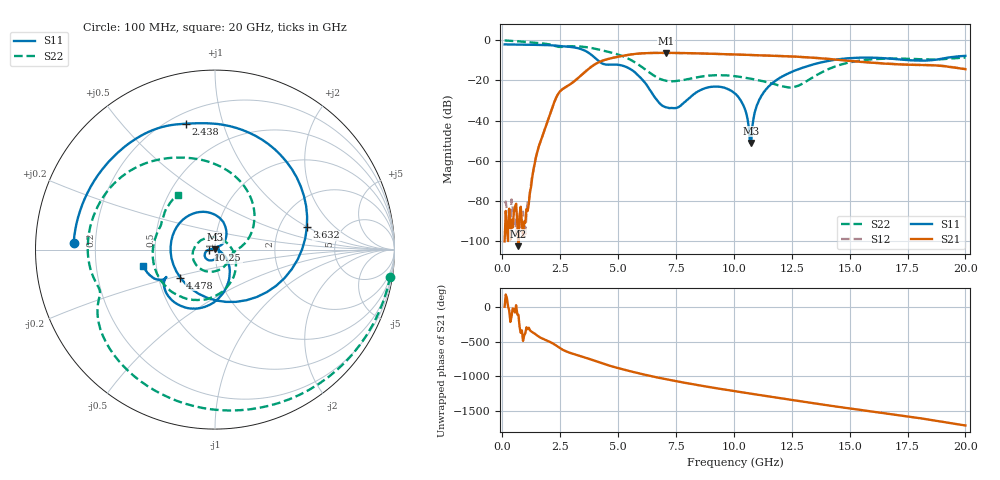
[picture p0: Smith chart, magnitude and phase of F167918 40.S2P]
!  2-Port S-parameters saved by WinCal
! VAR MeasName=S-Parameters (CALIBRATED_DATA) read from VNA (N5242A)
! VAR MeasDate=2016-11-22 10:26:40
! VAR NAME=F167918 40
! VAR FILENAME=F167918 40.S2P
! VAR DATE=2016-11-22 10:26:40
! VAR PHYS_PORTS=1,2
# Hz S DB R 50
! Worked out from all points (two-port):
!   401 points, 100 MHz to 20 GHz, reference 50 ohm
!   highest |S21| = -6.27 dB at 7.065 GHz (marker M1); lowest = -102.4 dB at 697 MHz (marker M2)
!   |S21| within 3 dB of the highest: 4.585 GHz to 14.08 GHz (9.496 GHz wide, 102 % of centre)
!   lowest |S11| = -51.1 dB at 10.75 GHz (marker M3), VSWR 1.01, Z = 50.2 + j0.14 ohm
!   |S11| at or under -10 dB: 4.123 GHz to 14.21 GHz (10.09 GHz wide, 110 % of centre); 17.69 GHz to 18.46 GHz (766.7 MHz wide, 4.24 % of centre)
!   |S22| runs from -23.5 to -0.1 dB; largest |S21 - S12| = 0.0056
!   S11 on the Smith chart (normalised r, x): 100 MHz: 0.12, +0.02; 2.438 GHz: 0.26, +0.76; 3.632 GHz: 2.85, +0.98; 4.478 GHz: 0.65, -0.22; 10.25 GHz: 0.93, -0.00; 20 GHz: 0.42, -0.10
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1e8  -2.07 177.3  -100.04 9.3  -81.12 -175.3  -0.10 -8.7
6.97e8  -2.15 161.4  -102.41 -107.9  -90.27 120.7  -0.53 -56.1
1.14475e9  -2.23 148.9  -81.33 65.2  -79.32 11.6  -0.96 -87.9
1.54275e9  -2.32 137.0  -54.26 -56.5  -54.14 -55.1  -1.37 -113.2
2.43825e9  -2.85 102.9  -26.24 140.6  -26.23 140.3  -3.30 -159.4
3.43325e9  -4.53 36.4  -17.17 6.7  -17.20 6.7  -3.19 157.2
3.63225e9  -5.57 13.6  -15.14 -14.7  -15.15 -14.6  -3.44 147.1
4.08e9  -9.57 -58.1  -11.45 -66.5  -11.41 -66.4  -4.41 124.8
4.478e9  -12.10 -140.9  -9.62 -110.9  -9.57 -111.1  -5.49 106.1
5.473e9  -13.96 93.7  -7.20 157.5  -7.22 157.2  -9.32 53.1
6.7665e9  -31.01 41.7  -6.28 57.2  -6.30 57.1  -19.01 -4.3
7.065e9  -33.36 46.1  -6.27 37.0  -6.30 37.0  -20.13 -13.3
8.70675e9  -24.09 -106.6  -6.59 -63.6  -6.59 -63.7  -17.87 -104.7
1.005e10  -26.50 -170.6  -7.08 -137.3  -7.09 -137.3  -17.90 -167.3
1.0249e10  -29.15 -178.9  -7.17 -147.8  -7.16 -147.7  -18.17 -174.5
1.07465e10  -51.13 30.2  -7.34 -173.6  -7.34 -173.6  -19.14 168.4
1.099525e10  -32.31 -16.6  -7.43 173.6  -7.41 173.6  -19.77 159.5
1.149275e10  -23.07 -34.5  -7.60 148.0  -7.59 148.0  -21.12 139.3
1.338325e10  -12.17 -79.3  -8.66 51.3  -8.59 51.5  -18.65 -18.0
1.67165e10  -9.12 -144.1  -11.69 -107.0  -11.69 -107.4  -9.11 -158.7
1.83085e10  -10.10 -150.4  -12.40 176.5  -12.26 175.9  -9.51 162.4
2e10  -7.74 -166.8  -14.38 85.3  -14.31 84.6  -8.64 124.4
